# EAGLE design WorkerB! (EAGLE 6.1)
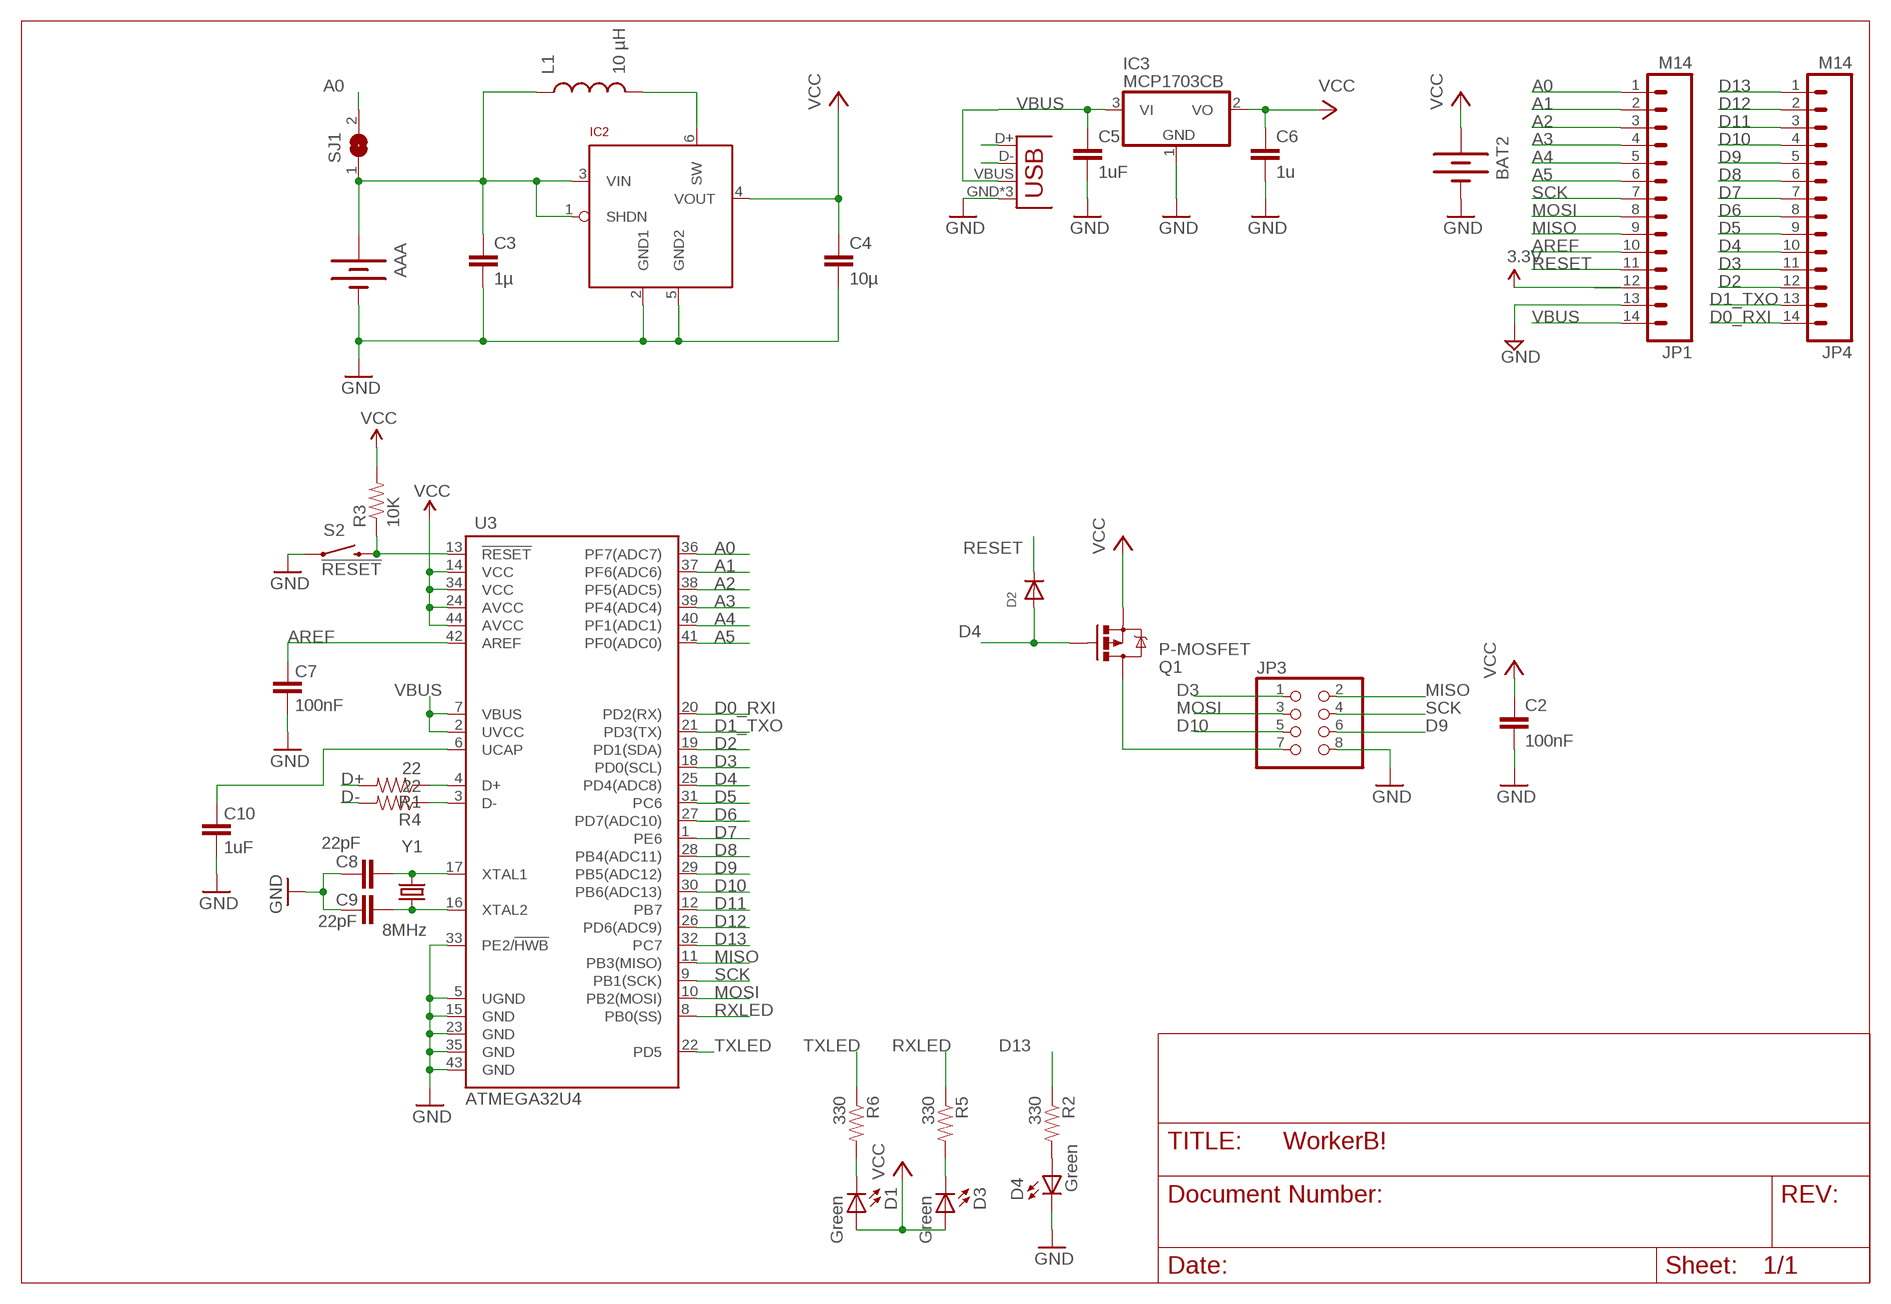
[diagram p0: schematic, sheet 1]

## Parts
AAA  BATTERYAAA-JL  [BATTERY-AAA-JL]
BAT2  BATTERY20PTH  [BATTCOM_20MM_PTH]
C2  100nF  C-EUC0603K  [C0603K]
C3  1µ  CAP0603-CAP  [0603-CAP]
C4  10µ  CAP0805  [0805]
C5  1uF  C-EUC0603K  [C0603K]
C6  1u  C-EUC0603K  [C0603K]
C7  100nF  CAP0402-CAP  [0402-CAP]
C8  22pF  CAP0402-CAP  [0402-CAP]
C9  22pF  CAP0402-CAP  [0402-CAP]
C10  1uF  CAP0402-CAP  [0402-CAP]
D1  Green  LED0603  [LED-0603]
D2  DIODESOD-323F  [SOD-323F]
D3  Green  LED0603  [LED-0603]
D4  Green  LED0603  [LED-0603]
IC2  LTC3525  [SC70]
IC3  MCP1703CB  [SOT23]
JP1  M14  [1X14]
JP2  USB-MICROB  [USB-MICROB]
JP3  PINHD-2X4  [2X04]
JP4  M14  [1X14]
L1  10 µH  INDUCTOR1210  [1210]
Q1  P-MOSFET  MOSFET-PCHANNEL  [SOT23]
R1  22  RESISTOR0402-RES  [0402-RES]
R2  330  RESISTOR0402-RES  [0402-RES]
R3  10K  RESISTOR0402-RES  [0402-RES]
R4  22  RESISTOR0402-RES  [0402-RES]
R5  330  RESISTOR0402-RES  [0402-RES]
R6  330  RESISTOR0402-RES  [0402-RES]
S2  !RESET  SWITCH-MOMENTARY-2SMD  [TACTILE_SWITCH_SMD]
SJ1  SJ  [SJ]
U3  ATMEGA32U4  ATMEGA32U4QFN2  [QFN-44-NOPAD]
Y1  8MHz  CRYSTAL5X3  [CRYSTAL-SMD-5X3]

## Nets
A0: JP1.1 SJ1.2 U3.36(PF7(ADC7))
A1: JP1.2 U3.37(PF6(ADC6))
A2: JP1.3 U3.38(PF5(ADC5))
A3: JP1.4 U3.39(PF4(ADC4))
A4: JP1.5 U3.40(PF1(ADC1))
A5: JP1.6 U3.41(PF0(ADC0))
AREF: C7.2 JP1.10 U3.42(AREF)
D0_RXI: JP4.14 U3.20(PD2(RX))
D1_TXO: JP4.13 U3.21(PD3(TX))
D2: JP4.12 U3.19(PD1(SDA))
D3: JP3.1 JP4.11 U3.18(PD0(SCL))
D4: D2.A JP4.10 Q1.1(G) U3.25(PD4(ADC8))
D5: JP4.9 U3.31(PC6)
D6: JP4.8 U3.27(PD7(ADC10))
D7: JP4.7 U3.1(PE6)
D8: JP4.6 U3.28(PB4(ADC11))
D9: JP3.6 JP4.5 U3.29(PB5(ADC12))
D10: JP3.5 JP4.4 U3.30(PB6(ADC13))
D11: JP4.3 U3.12(PB7)
D12: JP4.2 U3.26(PD6(ADC9))
D13: JP4.1 R2.1 U3.32(PC7)
D+: JP2.D+ R1.2
D-: JP2.D- R4.2
GND [power]: AAA.GND@1(-) BAT2.2(-) C2.2 C3.2 C4.2 C5.2 C6.2 C7.1 C8.2 C9.2 C10.1 D4.C IC2.2(GND1) IC2.5(GND2) IC3.1(GND) JP1.13 JP2.GND JP2.MT1(GND) JP2.MT2(GND) JP3.8 S2.1 U3.5(UGND) U3.15(GND) U3.23(GND) U3.33(PE2/!HWB) U3.35(GND) U3.43(GND)
MISO: JP1.9 JP3.2 U3.11(PB3(MISO))
MOSI: JP1.8 JP3.3 U3.10(PB2(MOSI))
N$1: C9.1 U3.16(XTAL2) Y1.1
N$2: R1.1 U3.4(D+)
N$3: D4.A R2.2
N$4: C8.1 U3.17(XTAL1) Y1.3
N$5: C10.2 U3.6(UCAP)
N$6: D3.C R5.2
N$7: R4.1 U3.3(D-)
N$8: D1.C R6.2
N$10: JP3.7 Q1.3(D)
N$13 [power]: IC2.6(SW) L1.2
RESET: D2.C JP1.11 R3.1 S2.3 U3.13(!RESET)
RXLED: R5.1 U3.8(PB0(SS))
SCK: JP1.7 JP3.4 U3.9(PB1(SCK))
TXLED: R6.1 U3.22(PD5)
VBUS [power]: C5.1 IC3.3(VI) JP1.14 JP2.VBUS U3.2(UVCC) U3.7(VBUS)
VCC [power]: BAT2.1(+) C2.1 C4.1 C6.1 D1.A D3.A IC2.4(VOUT) IC3.2(VO) JP1.12 Q1.2(S) R3.2 U3.14(VCC) U3.24(AVCC) U3.34(VCC) U3.44(AVCC) ; supply symbol labelled 3.3V
VIN: AAA.PWR@1(+) C3.1 IC2.1(SHDN) IC2.3(VIN) L1.1 SJ1.1

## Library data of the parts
AAA = JeeLabs:BATTERY: Battery Holders
BAT2 = SparkFun:BATTERY: Battery Holders
C2 C5 C6 = rcl:C-EU: CAPACITOR, European symbol
C3 C4 C7-C10 = SparkFun:CAP: Capacitor
D1 D3 D4 = SparkFun:LED: LEDs
D2 = adafruit:DIODE: Diode
IC2 = JeeLabs:LTC3525
IC3 = linear:MCP1703: 250 mA, 16V, Low Quiescent Current LDO Regulator Source: http://ww1.microchip.com/downloads/en/DeviceDoc/22049b.pdf
JP1 JP4 = SparkFun-Connectors:M14: Header 14 Standard 14-pin 0.1" header. Use with straight break away headers (SKU : PRT-00116), right angle break away headers (PRT-00553), swiss pins (PRT-00743), machine pins (PRT-00117), and female headers (PRT-00115).
JP2 = SparkFun-Connectors:USB: USB Connectors USB-B-PTH is fully proven SKU : PRT-00139/CONN-08278 USB-miniB is fully proven SKU : PRT-00587 USB-A-PCB is untested. USB-A-H is throughly reviewed, but untested. Spark Fun Electronics SKU : PRT-00437 USB-B-SMT is throughly reviewed, but untested. Needs silkscreen touching up.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; PROD_ID: CONN-09505
JP3 = pinhead:PINHD-2X4: PIN HEADER
L1 = SparkFun:INDUCTOR: Inductors
Q1 = SparkFun:MOSFET-PCHANNEL
R1-R6 = SparkFun:RESISTOR: Resistor
S2 = SparkFun-Electromechanical:SWITCH-MOMENTARY-2: Various NO switches- pushbuttons, reed, etc; PROD_ID: SWCH-08247
SJ1 = jumper:SJ: SMD solder JUMPER
U3 = SparkFun:ATMEGA32U4
Y1 = SparkFun:CRYSTAL: Crystals

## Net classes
1 power: width 0.203 mm, clearance 0.152 mm

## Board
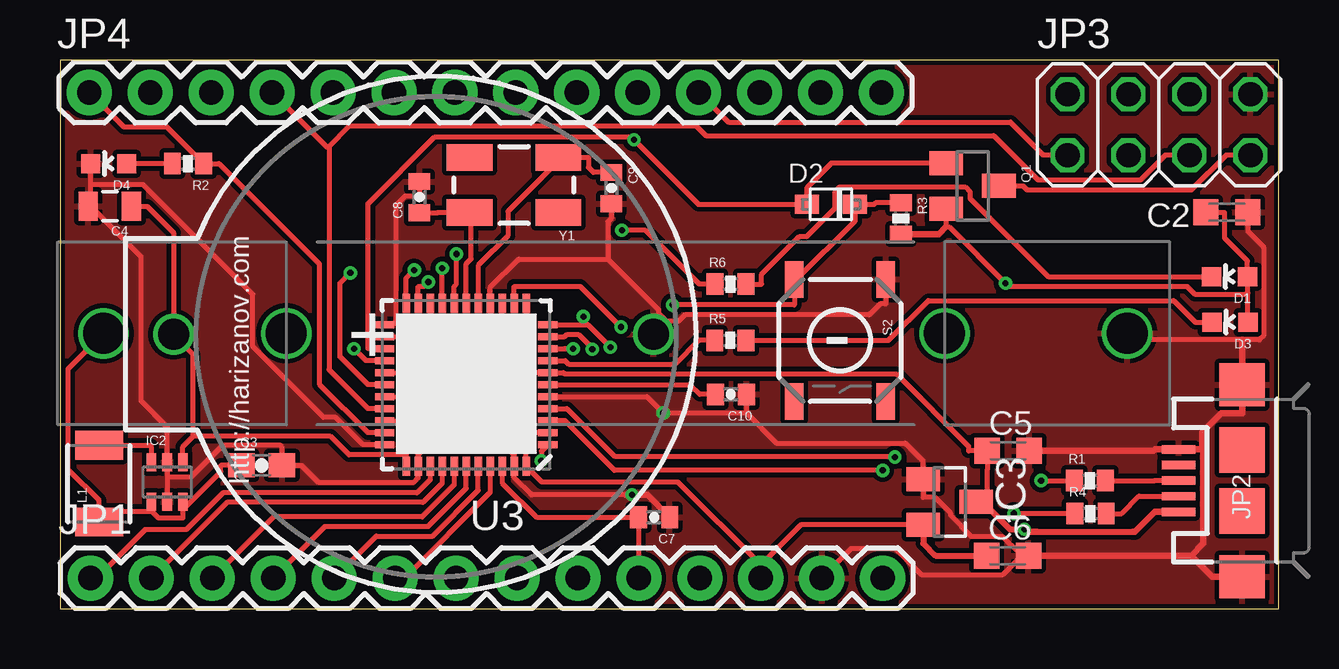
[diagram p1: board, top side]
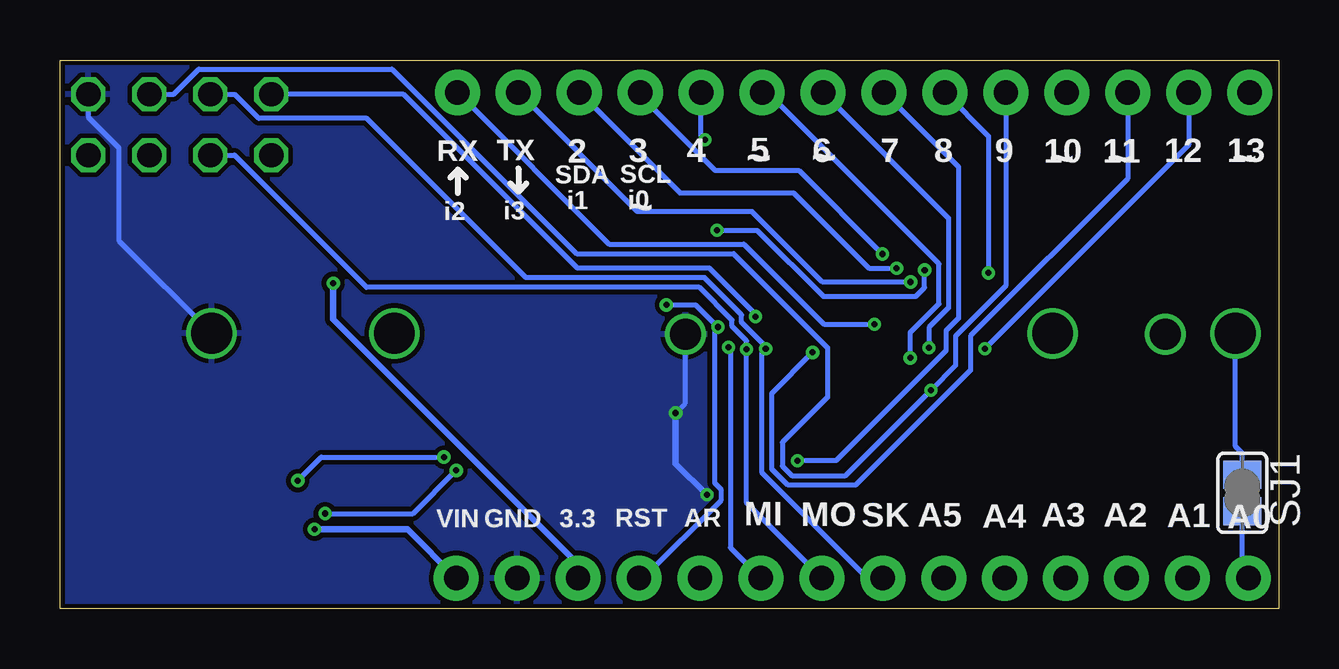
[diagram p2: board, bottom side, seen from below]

Size 50.81 x 22.86 mm. Coordinates in mm from the lower left corner, seen from the top.
Outline: 0,0 50.81,0 50.81,22.86 0,22.86 0,0
Copper layers (1*16): Top 0.035mm / dielectric 1.5mm / Bottom 0.035mm
Design rules: minimum track width 0.2mm, minimum drill 0.3mm, track to track 0.2mm, track to pad 0.2mm, pad to pad 0.2mm, via to via 0.2mm, smd to smd 0.2mm, copper to edge 0.2mm, drill to drill 0.2mm, minimum pad ring 0.2mm, minimum via ring 0.15mm, stop-mask expansion 0.075mm, vias tented up to drill 0.3mm, thermal gap 0.2mm

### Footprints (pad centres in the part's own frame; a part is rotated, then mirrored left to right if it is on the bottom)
BATTERY-AAA-JL = drill 1.702: GND@1 21.082,0; GND@2 13.462,0; PWR@1 -21.59,0; PWR@2 -13.97,0
BATTCOM_20MM_PTH = drill 1.3: 1 20,0; 2 0,0
C0603K = smd 1.05 x 1.08: 1 -0.875,0; 2 0.875,0
0603-CAP = smd 1.1 x 1: 1 -0.85,0; 2 0.85,0
0805 = smd 0.8 x 1.2: 1 -0.9,0; 2 0.9,0
0402-CAP = smd 0.7 x 0.9: 1 -0.65,0; 2 0.65,0
LED-0603 = smd 0.8 x 0.8: A 0,-0.75; C 0,0.75
SOD-323F = smd 1 x 0.8: A -1,0; C 1,0
SC70 = smd 0.4 x 0.75: 1 -0.65,-0.825; 2 0,-0.825; 3 0.65,-0.825; 4 0.65,0.825; 5 0,0.825; 6 -0.65,0.825
SOT23 = smd 1 x 1.4: 1 -0.95,-1.1; 2 0.95,-1.1; 3 0,1.1
1X14 = drill 1.016 pad 1.88: 1 0,0; 2 2.54,0; 3 5.08,0; 4 7.62,0; 5 10.16,0; 6 12.7,0; 7 15.24,0; 8 17.78,0; 9 20.32,0; 10 22.86,0; 11 25.4,0; 12 27.94,0; 13 30.48,0; 14 33.02,0
USB-MICROB = smd 0.35 x 1.4: D+ 0,2.65; D- -0.65,2.65; GND 1.3,2.65; ID 0.65,2.65; VBUS -1.3,2.65 | smd 1.8 x 1.9: MT1 -4,0; MT2 4,0 | smd 1.9 x 1.9: P$1 -1.27,0; P$2 1.27,0
2X04 = drill 1.016 octagon: 1 -3.81,-1.27; 2 -3.81,1.27; 3 -1.27,-1.27; 4 -1.27,1.27; 5 1.27,-1.27; 6 1.27,1.27; 7 3.81,-1.27; 8 3.81,1.27
1210 = smd 1.2 x 2: 1 -1.6,0; 2 1.6,0
0402-RES = smd 0.7 x 0.9: 1 -0.65,0; 2 0.65,0
TACTILE_SWITCH_SMD = smd 1.524 x 0.762: 1 -2.54,1.905; 2 2.54,1.905; 3 -2.54,-1.905; 4 2.54,-1.905
SJ = smd 1.168 x 1.6: 1 -0.762,0; 2 0.762,0
QFN-44-NOPAD = smd 0.8 x 0.3: 1 -3.4,2.5; 2 -3.4,2; 3 -3.4,1.5; 4 -3.4,1; 5 -3.4,0.5; 6 -3.4,0; 7 -3.4,-0.5; 8 -3.4,-1; 9 -3.4,-1.5; 10 -3.4,-2; 11 -3.4,-2.5; 23 3.4,-2.5; 24 3.4,-2; 25 3.4,-1.5; 26 3.4,-1; 27 3.4,-0.5; 28 3.4,0; 29 3.4,0.5; 30 3.4,1; 31 3.4,1.5; 32 3.4,2; 33 3.4,2.5 | smd 0.3 x 0.8: 12 -2.5,-3.4; 13 -2,-3.4; 14 -1.5,-3.4; 15 -1,-3.4; 16 -0.5,-3.4; 17 0,-3.4; 18 0.5,-3.4; 19 1,-3.4; 20 1.5,-3.4; 21 2,-3.4; 22 2.5,-3.4; 34 2.5,3.4; 35 2,3.4; 36 1.5,3.4; 37 1,3.4; 38 0.5,3.4; 39 0,3.4; 40 -0.5,3.4; 41 -1,3.4; 42 -1.5,3.4; 43 -2,3.4; 44 -2.5,3.4
CRYSTAL-SMD-5X3 = smd 1.9 x 1.1: 1 -1.85,-1.15; 2 1.85,-1.15; 3 1.85,1.15; 4 -1.85,1.15

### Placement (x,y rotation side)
AAA  23.4,11.47 0 top
BAT2  24.73,11.43 180 top
C2  48.64,16.51 0 top
C3  8.41,5.97 0 top
C4  2.08,16.76 180 top
C5  39.52,6.58 0 top
C6  39.5,2.21 0 top
C7  24.77,3.81 180 top
C8  14.99,17.14 90 top
C9  22.99,17.53 270 top
C10  27.97,8.93 180 top
D1  48.75,13.83 90 top
D2  32.14,16.85 0 top
D3  48.77,11.94 90 top
D4  2.03,18.54 90 top
IC2  4.47,5.28 0 top
IC3  37.08,4.45 270 top
JP1  1.27,1.27 0 top
JP2  49.28,5.33 90 top
JP3  45.81,20.16 0 top
JP4  1.22,21.51 0 top
L1  1.63,5.21 90 top
Q1  38.04,17.61 270 top
R1  42.93,5.33 0 top
R2  5.33,18.54 180 top
R3  35.05,16.26 270 top
R4  42.95,3.96 0 top
R5  27.94,11.18 0 top
R6  27.95,13.52 0 top
S2  32.51,11.18 270 top
SJ1  1.52,4.83 270 bottom
U3  16.94,9.33 180 top
Y1  18.92,17.65 180 top

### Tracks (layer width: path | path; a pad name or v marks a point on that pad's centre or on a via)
A0
  Top 0.2: U3.36 15.44,5.38 14.88,4.82 6.8,4.82 5.26,3.29 3.55,3.29 1.53,1.27 JP1.1
  Bottom 0.2: JP1.1 1.52,1.52 SJ1.2
A1
  Top 0.2: U3.37 15.94,5.23 15.13,4.42 6.96,4.42 JP1.2
A2
  Top 0.2: U3.38 16.43,5.16 15.1,3.82 8.9,3.82 JP1.3
A3
  Top 0.2: JP1.4 11.04,3.42 15.35,3.42 16.93,5.01 U3.39
A4
  Top 0.2: JP1.5 13.18,3.02 15.53,3.02 17.43,4.92 U3.40
A5
  Top 0.2: U3.41 17.93,4.85 14.36,1.27 JP1.6
AREF
  Top 0.2: U3.42 18.43,5.23 19.86,3.81 C7.2 24.11,1.28 JP1.10
D0_RXI  (via drill 0.25 pad 0.55)
  Top 0.2: v16.86,11.85 16.68,12.03 15.44,12.03 U3.20
  Bottom 0.2: JP4.14 27.92,15.19 22.3,15.19 18.96,11.85 v16.86,11.85
D1_TXO  (via drill 0.25 pad 0.55)
  Top 0.2: U3.21 14.94,13.43 15.17,13.43 v15.35,13.61
  Bottom 0.2: v15.35,13.61 19.02,13.61 21.96,16.55 26.74,16.55 JP4.13
D2  (via drill 0.25 pad 0.55)
  Top 0.2: U3.19 v15.94,14.19
  Bottom 0.2: JP4.12 24.97,17.32 20.22,17.32 17.09,14.19 v15.94,14.19
D3  (via drill 0.25 pad 0.55)
  Top 0.2: U3.18 16.43,13.43 16.53,13.52 v16.53,14.78 | JP3.1 40.99,18.89 39.62,20.27 27.86,20.27 JP4.11
  Bottom 0.2: JP4.11 26.62,21.39 23.5,18.26 20.01,18.26 v16.53,14.78
D4  (via drill 0.25 pad 0.55)
  Top 0.2: Q1.1 32.15,18.56 31.14,17.55 D2.A 26.61,16.85 v23.92,19.54 23.81,19.65 15.62,19.65 12.84,16.87 12.84,10.83 U3.25
  Bottom 0.2: v23.92,19.54 24.08,19.69 JP4.10
D5  (via drill 0.25 pad 0.55)
  Top 0.2: U3.31 14.23,7.83 15.37,8.96 v15.37,10.45
  Bottom 0.2: v15.37,10.45 15.37,11.51 14.17,12.7 14.17,14.37 21.31,21.51 JP4.9
D6  (via drill 0.25 pad 0.55)
  Top 0.2: U3.27 14.23,9.83 14.23,10.52 v14.59,10.87
  Bottom 0.2: JP4.8 13.77,16.28 13.77,12.54 14.59,11.72 v14.59,10.87
D7  (via drill 0.25 pad 0.55)
  Top 0.2: U3.1 20.06,6.56 v20.06,6.17
  Bottom 0.2: JP4.7 13.36,18.41 13.36,12.1 13.87,11.58 13.87,10.75 18.46,6.17 v20.06,6.17
D8  (via drill 0.25 pad 0.55)
  Top 0.2: U3.28 12.84,9.33 11.68,10.49 11.68,13.56 v12.1,13.99
  Bottom 0.2: JP4.6 12.1,19.69 v12.1,13.99
D9  (via drill 0.25 pad 0.55)
  Top 0.2: U3.29 14.23,8.83 v14.51,9.1
  Bottom 0.2: JP3.6 46.07,21.43 45.02,22.48 36.97,22.48 29.27,14.79 22.73,14.79 18.82,10.88 18.82,8.81 20.69,6.93 20.69,5.94 20.3,5.54 18.07,5.54 v14.51,9.1 13.47,10.13 13.47,11.36 11.38,13.45 JP4.5
D10
  Top 0.2: 11.21,19.24 12.08,20.11 26.52,20.11 26.92,19.71 38.92,19.71 40.77,17.86 45.04,17.86 46.07,18.89 JP3.5 | JP4.4 11.11,19.24 11.21,19.24 | 11.21,19.24 11.21,9.96 12.84,8.33 U3.30
D11  (via drill 0.25 pad 0.55)
  Top 0.2: U3.12 v19.43,10.68
  Bottom 0.2: JP4.3 6.3,17.91 12.85,11.36 12.85,9.93 17.64,5.14 20.46,5.14 21.14,5.82 21.14,8.97 v19.43,10.68
D12  (via drill 0.25 pad 0.55)
  Top 0.2: U3.26 12.75,10.33 v12.25,10.83
  Bottom 0.2: JP4.2 3.76,19.32 v12.25,10.83
D13
  Top 0.2: U3.32 12.84,7.33 10.81,9.36 10.81,14.37 6.63,18.54 R2.1 4.47,20.06 2.67,20.06 JP4.1
D+
  Top 0.2: R1.2 45.63,5.33 JP2.D+
D-
  Top 0.2: R4.2 44.25,3.96 44.97,4.68 JP2.D-
GND  (via drill 0.25 pad 0.55)
  Top 0.2: 28.62,8.15 v25.14,8.15 24.46,8.83 U3.5
  Top 0.203: 23.58,4.74 19.65,4.74 18.93,5.46 U3.43 18.93,6.42 18.72,6.63 15.15,6.63 14.94,6.42 U3.35 14.94,5.45 14.76,5.28 10.76,5.28 10.06,5.97 C3.2 9.26,6.72 9.17,6.81 6.78,6.81 5.45,5.48 4.47,5.48 | 22.84,14.57 24.95,12.46 24.95,12.31 25.28,11.98 | 22.84,14.57 19.12,14.57 17.93,13.38 U3.15 17.93,12.08 17.11,11.26 15.88,11.26 15.75,11.38 15.43,11.38 14.86,11.95 13.98,11.95 | 22.84,14.57 22.84,16.12 22.99,16.27 C9.2 | 25.28,11.98 25.78,11.98 26.05,12.24 33.74,12.24 34.19,12.69 34.41,12.69 34.42,12.7 S2.1 | 25.28,11.98 | BAT2.2 25.28,11.98 | AAA.GND@1 44.62,11.33 44.76,11.2 49.28,11.2 49.99,11.2 50.17,11.38 50.17,15.06 49.52,15.72 C2.2 | 13.98,11.95 13.87,11.83 U3.23 | 13.98,11.95 13.98,16.79 14.38,17.19 14.99,17.19 C8.2 | 40.18,2.21 39.98,2.21 | C4.2 1.28,16.76 | C10.1 28.62,8.15 29.87,6.89 35.24,6.89 35.98,6.15 IC3.1 35.98,4.64 36.46,4.64 37.13,3.97 37.13,3.88 38.01,3 39.29,3 39.98,2.31 39.98,2.21 | 4.47,5.48 IC2.5 4.47,7.56 3.38,8.65 3.38,14.67 1.28,16.76 | 4.47,5.48 IC2.2 | 1.28,16.76 1.28,17.67 | 1.28,17.67 D4.C | JP1.13 32.99,2.51 34.82,2.51 35.91,1.42 39.3,1.42 39.98,2.1 39.98,2.21 | U3.33 12.63,6.83 11.49,7.97 10.98,7.97 8.03,10.92 8.03,13.1 3.47,17.67 1.28,17.67
  Top 0.279: C7.1 24.48,4.74 v23.84,4.74 23.58,4.74 | C5.2 45.58,6.58 45.63,6.63 JP2.GND 47.62,6.63 | 47.16,2.21 48.03,1.33 JP2.MT1 | 47.16,2.21 C6.2 40.18,2.21 | 47.62,6.63 47.67,6.59 47.67,2.72 47.16,2.21 | 47.62,6.63 47.62,7.36 48.4,8.14 49.28,8.14 JP2.MT2 49.28,11.2
  Bottom 0.203: v25.14,8.15 24.73,8.56 BAT2.2 | JP3.8 49.62,20.47 48.35,19.2 48.35,15.33 AAA.GND@1
  Bottom 0.279: v23.84,4.74 25.14,6.04 v25.14,8.15
  pour Bottom: 0,22.86 50.8,22.86 50.8,0 0,0
  pour Top: 0,22.86 50.8,22.86 50.8,0 0,0
MISO  (via drill 0.25 pad 0.55)
  Top 0.2: 21.82,11.83 22,11.83 v22.94,10.89 | U3.11 21.82,11.83 | 21.82,11.83 v21.82,12.17
  Bottom 0.2: v21.82,12.17 21.82,12.27 23.74,14.19 29.24,14.19 36.48,21.43 JP3.2 | v22.94,10.89 22.86,10.81 22.86,2.54 JP1.9
MOSI  (via drill 0.25 pad 0.55)
  Top 0.2: U3.10 21.04,11.33 21.11,11.41 21.63,11.41 22.19,10.85 v22.19,10.81
  Bottom 0.2: JP3.3 43.53,18.89 38.03,13.39 24.16,13.39 22.8,12.02 22.8,11.76 22.19,11.16 v22.19,10.81 22.19,4.41 JP1.8
N$1
  Top 0.2: 20.92,18.8 18.67,16.55 18.67,15.54 17.43,14.3 U3.16 | 20.92,18.8 22.02,18.8 22.02,18.39 22.24,18.18 C9.1 | Y1.1 20.92,18.8
N$2  (via drill 0.25 pad 0.55)
  Top 0.2: v40.89,5.33 R1.1 | U3.4 21.13,8.33 23.11,6.35 34.77,6.35 v34.8,6.32
  Bottom 0.2: v40.89,5.33 39.91,6.32 v34.8,6.32
N$3
  Top 0.2: R2.2 D4.A
N$4
  Top 0.2: U3.17 16.93,14.37 17.14,14.58 17.14,16.43 Y1.3 15.74,16.5 C8.1
N$5
  Top 0.2: U3.6 26.27,9.33 26.67,8.93 C10.2
N$6
  Top 0.2: R5.2 34.54,11.18 36.19,12.83 46.42,12.83 47.32,11.94 D3.C
N$7  (via drill 0.25 pad 0.55)
  Top 0.2: R4.1 v39.76,3.96 | v34.29,5.76 23.11,5.76 21.04,7.83 U3.3
  Bottom 0.2: v39.76,3.96 36.09,3.96 v34.29,5.76
N$8
  Top 0.2: R6.2 29.25,13.52 29.25,13.93 30.82,15.51 31.13,15.51 32.31,16.69 32.31,17.37 32.51,17.57 37.74,17.57 37.94,17.37 37.94,17.09 41.19,13.83 D1.C
N$10
  Top 0.2: JP3.7 48.61,18.89 47.17,17.45 40.3,17.45 40.14,17.61 Q1.3
N$13
  Top 0.203: IC2.6 3.82,6.74 3.75,6.81 L1.2
RESET  (via drill 0.25 pad 0.55)
  Top 0.2: v23.38,11.73 21.69,13.43 18.93,13.43 U3.13 | v25.53,12.65 30.61,12.65 S2.3 30.71,13.72 33.14,16.15 D2.C 33.94,16.85 34,16.91 R3.1
  Bottom 0.2: 23.52,11.73 23.52,5.24 23.26,4.98 23.26,4.5 26.5,1.27 JP1.11 | 23.52,11.73 v23.38,11.73 | v25.53,12.65 24.31,12.65 23.52,11.87 23.52,11.73
RXLED
  Top 0.2: U3.8 21.06,10.33 21.2,10.18 25.65,10.18 26.64,11.18 R5.1
SCK  (via drill 0.25 pad 0.55)
  Top 0.2: v21.39,10.83 21.04,10.83 U3.9
  Bottom 0.2: JP3.4 43.53,21.43 42.52,20.42 38.02,20.42 31.38,13.79 23.94,13.79 22.39,12.24 22.39,11.93 21.39,10.92 v21.39,10.83 21.54,10.68 21.54,5.66 17.16,1.27 JP1.7
TXLED  (via drill 0.25 pad 0.55)
  Top 0.2: v23.42,15.77 24.4,15.77 26.65,13.52 R6.1 | U3.22 14.44,13.78 v14.77,14.11
  Bottom 0.2: v23.42,15.77 21.75,15.77 18.99,13.01 15.13,13.01 14.77,13.38 v14.77,14.11
VBUS  (via drill 0.25 pad 0.55)
  Top 0.203: 38.65,4.45 38.65,4.25 | 40.2,3.21 40.33,3.21 | U3.2 19.68,7.33 19.63,7.38 19.63,9.78 19.68,9.83 U3.7 20.99,9.83 21.04,9.78 34.86,9.78 37.87,6.77 37.87,6.58 C5.1 38.65,5.79 38.65,4.45 | IC3.3 38.65,4.45
  Top 0.254: 38.65,4.25 39.59,3.31 v40.2,3.31 | 40.73,3.21 44.71,3.21
  Top 0.279: 40.2,3.21 v40.2,3.31 | 40.33,3.21 40.73,3.21 | JP2.VBUS 45.63,4.03 44.81,3.21 44.71,3.21
  Bottom 0.279: v40.2,3.31 36.33,3.31 JP1.14
VCC  (via drill 0.25 pad 0.55)
  Top 0.203: Q1.2 36.94,15.91 37.06,15.91 v39.41,13.56 | 39.41,13.43 46.98,13.43 47.3,13.11 49.42,13.11 49.5,13.18 | 29.21,1.82 25.76,5.27 20.09,5.27 U3.44 19.43,6.58 18,8.02 16.41,8.02 | 16.41,10.21 15.6,11.03 15.26,11.03 14.82,11.46 14.32,11.46 14.19,11.33 U3.24 | 16.41,8.02 16.41,10.21 | 16.41,10.21 16.58,10.21 18.43,12.07 U3.14 | C2.1 48.55,16.51 48.55,15.44 49.5,14.49 D1.A 49.5,13.18 | D3.A 49.52,13.16 49.5,13.18 | IC3.2 30.88,3.5 29.21,1.82 | C4.1 3.64,16.76 4.73,15.67 BAT2.1 5.56,10.61 5.56,7.18 | 29.21,1.82 JP1.12 | IC2.4 5.12,6.74 5.56,7.18 | 16.41,8.02 15.96,8.02 14.44,6.5 14.44,6.41 | 14.44,6.41 U3.34 | 14.44,6.41 12.05,6.41 11.28,7.18 5.56,7.18
  Top 0.254: IC3.2 35.98,2.72 36.49,2.21 C6.1
  Top 0.279: R3.2 36.63,15.61 36.94,15.91 | v39.41,13.56 39.41,13.43
  Bottom 0.279: JP1.12 29.21,1.84 39.41,12.05 v39.41,13.56 | v39.41,13.56
VIN
  Top 0.2: C3.1 6.71,5.97 6.71,5.71 5.12,4.12 | 5.12,4.12 5.12,3.78 4.09,3.78 3.82,4.06 | IC2.3 5.12,4.12 | 1.63,4.06 3.82,4.06 | IC2.1 3.82,4.06 | 1.63,4.06 1.63,4.51 0.33,5.81 0.33,9.98 AAA.PWR@1 | L1.1 1.63,4.06
  Bottom 0.2: SJ1.1 1.52,6.47 1.81,6.76 AAA.PWR@1

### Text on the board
tPlace: http://harizanov.com
_bsilk: 13 | 12 | 11 | 10 | 9 | 8 | 7 | 6 | 5 | 4 | 3 | 2 | TX | RX | ~ | ~ | ~ | ~ | ~ | SCL | SDA | i0 | i1 | ~ | i3 | i2 | AR | RST | GND | A0 | A1 | A2 | A3 | A4 | A5 | SK | MO | MI | 3.3 | VIN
